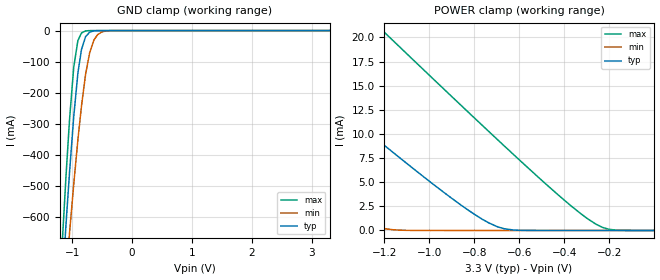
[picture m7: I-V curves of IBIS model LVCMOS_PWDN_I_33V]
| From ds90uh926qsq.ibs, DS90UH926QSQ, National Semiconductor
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[Model] LVCMOS_PWDN_I_33V
Model_type Input
Vinh = 2.0V
Vinl = 0.8V
C_comp   6.98pF   6.05pF   8.06pF
[Voltage Range]   3.3V   2.97V   3.63V
[Temperature Range]   25.0   130.0   -40.0
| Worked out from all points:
|   GND clamp passes 1 mA (typ) near -0.64 V on its own axis
|   POWER clamp passes 1 mA (typ) near -0.75 V on its own axis
[GND Clamp]
-3.3V     -7.729A    -6.4A      -8.658A
-1.171V   -833.9mA   -960.9mA   -705.2mA
-1.102V   -623.3mA   -790.6mA   -467.6mA
-1.043V   -454.3mA   -650.1mA   -284.8mA
-973.5mV  -277.4mA   -494.8mA   -117.8mA
-904.2mV  -136.9mA   -352.1mA   -32.17mA
-844.8mV  -61.17mA   -243.7mA   -7.849mA
-775.5mV  -19.32mA   -140.4mA   -1mA
-706.2mV  -4.954mA   -70.01mA   -73.86uA
-636.9mV  -976.4uA   -30.5mA    -9.519uA
-438.9mV  -7.484uA   -1.422mA   -4.418uA
3.293V    2.153uA    0A         3.15uA
[POWER Clamp]
-3.3V     49.92mA    32.15mA    67.97mA
-2.597V   36.03mA    20.71mA    52.03mA
-1.835V   21.07mA    8.533mA    34.8mA
-1.795V   20.29mA    7.917mA    33.91mA
-1.399V   12.62mA    2.096mA    25mA
-1.201V   8.843mA    191.4uA    20.57mA
-864.6mV  2.719mA    2.197uA    13.09mA
-696.3mV  375.1uA    1.956uA    9.394mA
-399.3mV  2.753uA    1.623uA    3.116mA
-260.7mV  2.512uA    1.496uA    662.9uA
-201.3mV  2.422uA    1.447uA    116.6uA
-3.3mV    2.164uA    1.307uA    3.559uA
